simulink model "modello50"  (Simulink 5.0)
settings: Solver=ode45  StartTime=0.0  StopTime=200  RelTol=1e-3
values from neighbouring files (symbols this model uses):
  Ct = Ctfe+Ctcu    [Capacita.m]
  DTreg = 49.3    [Capacita.m]    (also in limit.m; Raffred.m; Riscald.m)
  Gt = 1/Rt    [Capacita.m]
  Pp = DTreg/Rt    [Capacita.m]

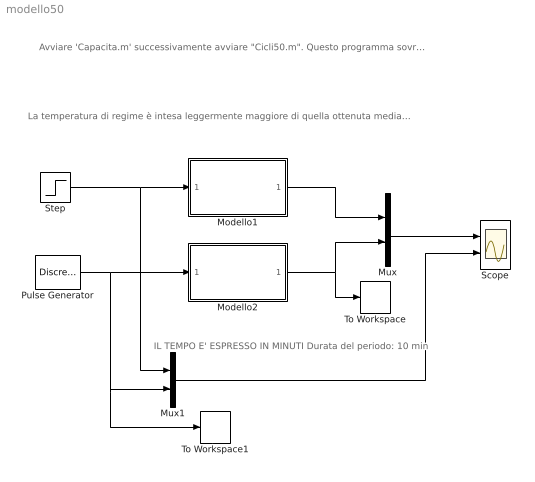
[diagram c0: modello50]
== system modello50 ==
  note: IL TEMPO E' ESPRESSO IN MINUTI Durata del periodo: 10 min
  note: Avviare 'Capacita.m' successivamente avviare "Cicli50.m". Questo programma sovrappone i risultati delle misure con quelli ottenuti con il modello.
  note: La temperatura di regime è intesa leggermente maggiore di quella ottenuta mediante il fitting dei dati del riscaldamento, e comunque il valore è gestito dal programma "Capacita.m"
  Modello1 : Subsystem
  Modello2 : Subsystem
  Mux : Mux  Inputs=2
  Mux1 : Mux  Inputs=2
  Pulse Generator : DiscretePulseGenerator  PulseType=Time based  Amplitude=2*Pp  Period=10  PulseWidth=50  PhaseDelay=5  SampleTime=10
  Scope : Scope  NumInputPorts=2
  Step : Step  Time=0  After=Pp  SampleTime=0
  To Workspace : ToWorkspace  VariableName=c50  SampleTime=-1  SaveFormat=Array
  To Workspace1 : ToWorkspace  VariableName=pulse  SampleTime=-1  SaveFormat=Array
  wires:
  Step/1 -> Modello1/1(In1), Mux1/1
  Mux/1 -> Scope/1
  Modello1/1(Out1) -> Mux/1
  Pulse Generator/1 -> Modello2/1(In1), Mux1/2, To Workspace1/1
  Modello2/1(Out1) -> Mux/2, To Workspace/1
  Mux1/1 -> Scope/2

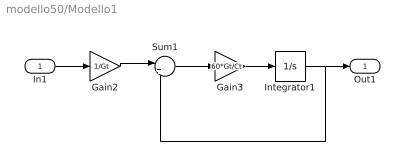
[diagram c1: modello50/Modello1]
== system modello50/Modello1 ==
  In1 : Inport
  Gain2 : Gain  Gain=1/Gt
  Gain3 : Gain  Gain=60*Gt/Ct
  Integrator1 : Integrator  InitialCondition=DTreg
  Sum1 : Sum  Inputs=|+-
  Out1 : Outport
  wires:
  Gain2/1 -> Sum1/1
  Sum1/1 -> Gain3/1
  Gain3/1 -> Integrator1/1
  Integrator1/1 -> Sum1/2, Out1/1
  In1/1 -> Gain2/1

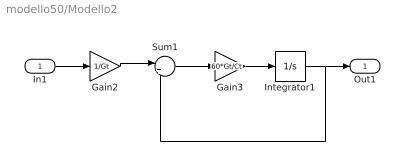
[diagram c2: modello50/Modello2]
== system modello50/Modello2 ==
  In1 : Inport
  Gain2 : Gain  Gain=1/Gt
  Gain3 : Gain  Gain=60*Gt/Ct
  Integrator1 : Integrator  InitialCondition=49.2
  Sum1 : Sum  Inputs=|+-
  Out1 : Outport
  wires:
  In1/1 -> Gain2/1
  Integrator1/1 -> Out1/1, Sum1/2
  Gain3/1 -> Integrator1/1
  Sum1/1 -> Gain3/1
  Gain2/1 -> Sum1/1
